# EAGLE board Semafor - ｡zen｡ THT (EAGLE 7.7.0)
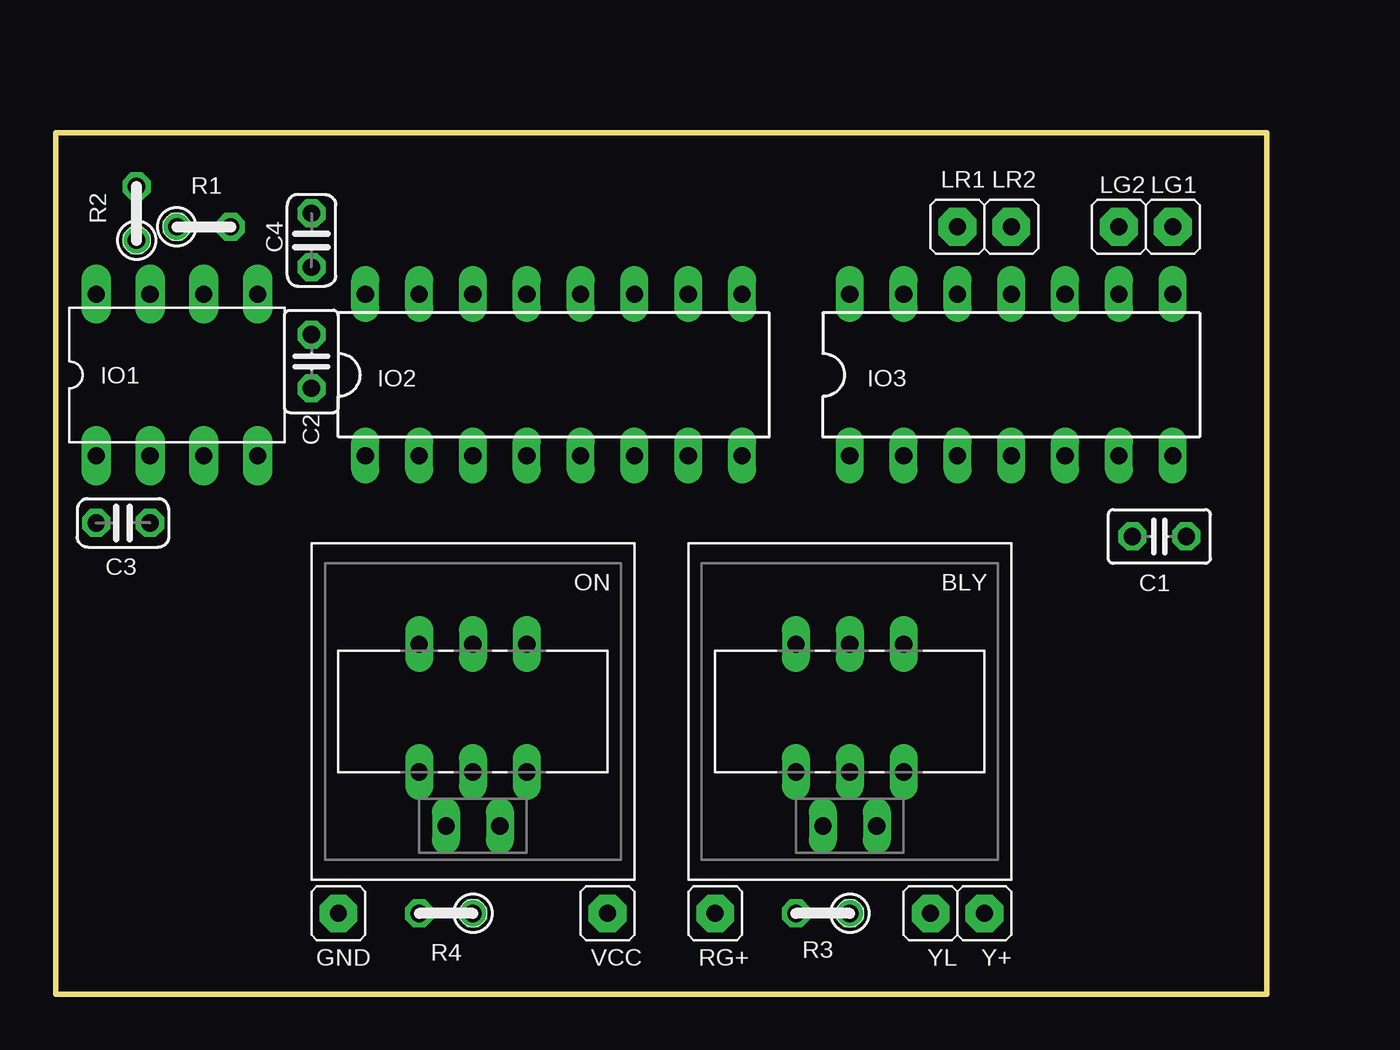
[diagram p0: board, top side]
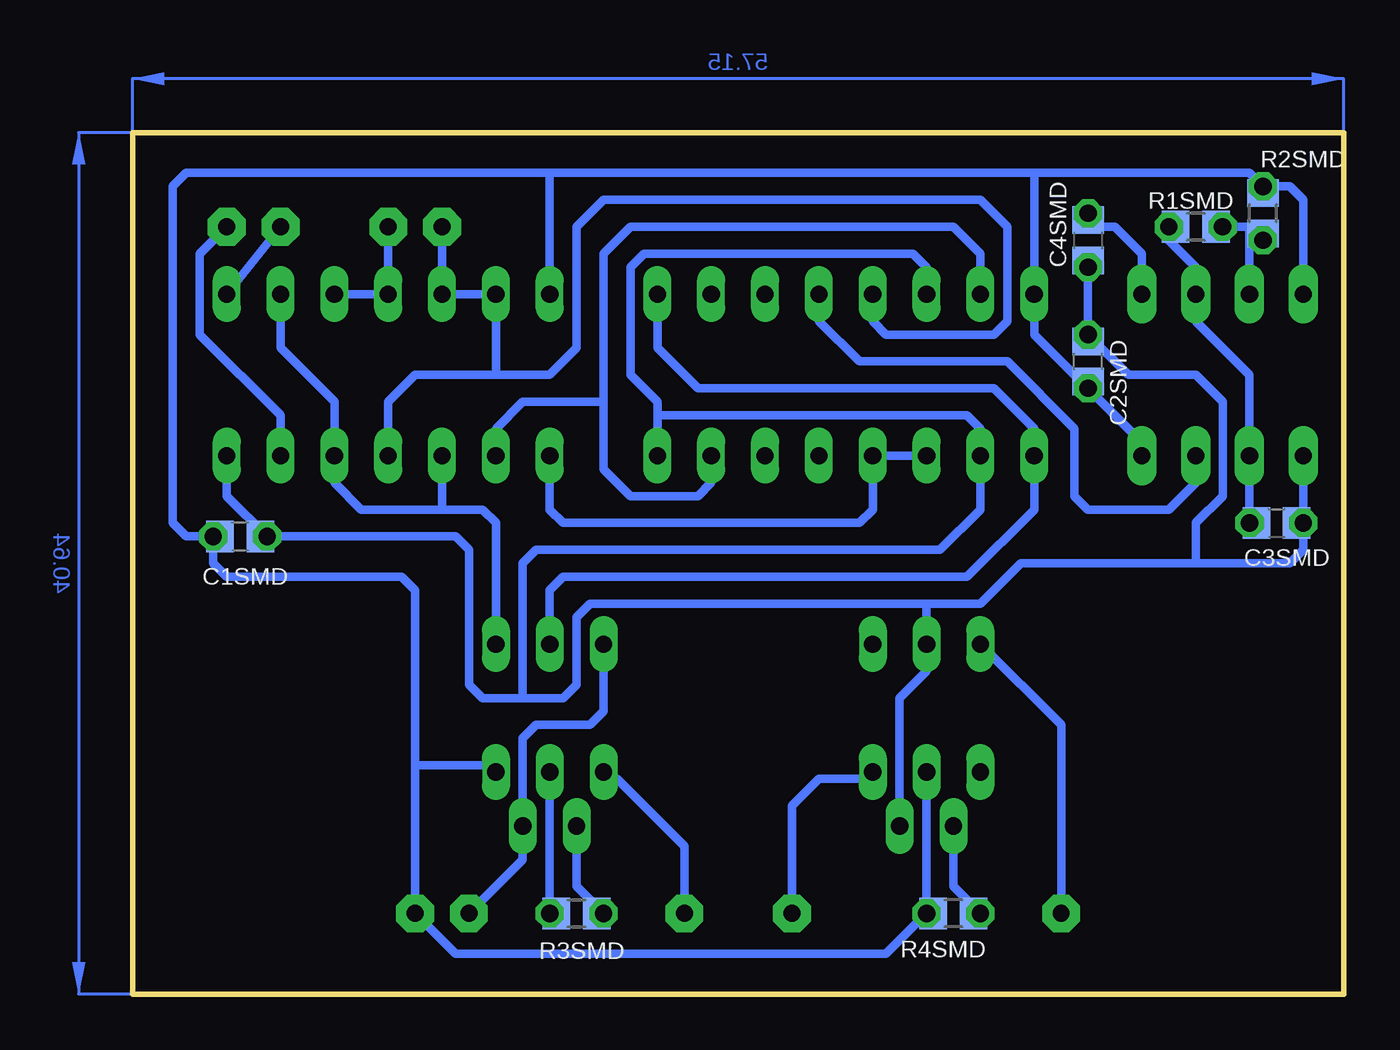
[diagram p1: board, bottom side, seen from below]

Size 57.15 x 40.64 mm. Coordinates in mm from the lower left corner, seen from the top.
Outline: 0,0 57.15,0 57.15,40.64 0,40.64 0,0
Copper layers (1*16): Top 0.035mm / dielectric 1.5mm / Bottom 0.035mm
Design rules "default": minimum track width 10mil, minimum drill 24mil, track to track 8mil, track to pad 8mil, pad to pad 8mil, via to via 8mil, smd to smd 8mil, copper to edge 40mil, drill to drill 8mil, minimum pad ring 10mil, minimum via ring 8mil, stop-mask expansion 4mil, vias tented up to drill 0mil, thermal gap 10mil

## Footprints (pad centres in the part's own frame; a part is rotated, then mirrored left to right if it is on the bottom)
P-0S?B = drill 0.813 pad 1.27 long: 1 2.54,-3.175; 2 0,-3.175; 3 -2.54,-3.175; 4 -2.54,2.857; 5 0,2.857; 6 2.54,2.857; A1 1.27,5.397; K1 -1.27,5.397
C025-025X050 = drill 0.813 octagon: 1 -1.27,0; 2 1.27,0
C0805 = smd 1.3 x 1.5: 1 -0.95,0; 2 0.95,0
C025-024X044 = drill 0.813 octagon: 1 -1.27,0; 2 1.27,0
S1G1_JUM = drill 0.8 pad 1.778 octagon: 1 0,0
DIL8 = drill 0.813 pad 1.4 long: 1 -3.81,-3.81; 2 -1.27,-3.81; 3 1.27,-3.81; 4 3.81,-3.81; 5 3.81,3.81; 6 1.27,3.81; 7 -1.27,3.81; 8 -3.81,3.81
DIL16 = drill 0.813 long: 1 -8.89,-3.81; 2 -6.35,-3.81; 3 -3.81,-3.81; 4 -1.27,-3.81; 5 1.27,-3.81; 6 3.81,-3.81; 7 6.35,-3.81; 8 8.89,-3.81; 9 8.89,3.81; 10 6.35,3.81; 11 3.81,3.81; 12 1.27,3.81; 13 -1.27,3.81; 14 -3.81,3.81; 15 -6.35,3.81; 16 -8.89,3.81
DIL14 = drill 0.813 long: 1 -7.62,-3.81; 2 -5.08,-3.81; 3 -2.54,-3.81; 4 0,-3.81; 5 2.54,-3.81; 6 5.08,-3.81; 7 7.62,-3.81; 8 7.62,3.81; 9 5.08,3.81; 10 2.54,3.81; 11 0,3.81; 12 -2.54,3.81; 13 -5.08,3.81; 14 -7.62,3.81
0204V = drill 0.813 octagon: 1 -1.27,0; 2 1.27,0
R0805 = smd 1.3 x 1.5: 1 -0.95,0; 2 0.95,0

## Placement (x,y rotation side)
BLY  [P-0S?B]  37.47,13.34 180 top
C1  [C025-025X050]  52.07,21.59 180 top
C1SMD  [C0805]  52.07,21.59 0 bottom
C2  [C025-025X050]  12.06,29.84 90 top
C2SMD  [C0805]  12.06,29.84 90 bottom
C3  [C025-024X044]  3.17,22.23 180 top
C3SMD  [C0805]  3.17,22.23 0 bottom
C4  [C025-024X044]  12.06,35.56 270 top
C4SMD  [C0805]  12.06,35.56 270 bottom
GND  [S1G1_JUM]  13.34,3.81 0 top
IO1  CMOS555  [DIL8]  5.71,29.21 0 top
IO2  74HCT390  [DIL16]  23.5,29.21 0 top
IO3  74HCT00  [DIL14]  45.09,29.21 0 top
LG1  [S1G1_JUM]  52.7,36.2 0 top
LG2  [S1G1_JUM]  50.16,36.2 0 top
LR1  [S1G1_JUM]  42.55,36.2 0 top
LR2  [S1G1_JUM]  45.09,36.2 0 top
ON  [P-0S?B]  19.68,13.34 180 top
R1  [0204V]  6.99,36.2 0 top
R1SMD  [R0805]  6.99,36.2 180 bottom
R2  [0204V]  3.81,36.83 90 top
R2SMD  [R0805]  3.81,36.83 90 bottom
R3  [0204V]  36.2,3.81 180 top
R3SMD  [R0805]  36.2,3.81 0 bottom
R4  [0204V]  18.41,3.81 180 top
R4SMD  [R0805]  18.41,3.81 180 bottom
RG+  [S1G1_JUM]  31.11,3.81 0 top
VCC  [S1G1_JUM]  26.04,3.81 0 top
Y+  [S1G1_JUM]  43.81,3.81 0 top
YL  [S1G1_JUM]  41.27,3.81 0 top

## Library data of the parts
BLY ON = #PaJa_prepinace
C1 C1SMD C2 C2SMD C3 C3SMD C4 C4SMD R1 R1SMD R2 R2SMD R3 R3SMD R4 R4SMD = rcl
GND LG1 LG2 LR1 LR2 RG+ VCC Y+ YL = #PaJa_konektory
IO1 = #PaJa_31
IO2 IO3 = 74xx-eu

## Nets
N$1: ON.A1 R4.2 R4SMD.1
N$2: BLY.6 RG+.1
N$4: GND.1 ON.1
N$5: ON.4 VCC.1
N$6: BLY.A1 R3.2 R3SMD.2
N$8: BLY.1 BLY.K1 YL.1
N$9: IO2.13 IO3.4 IO3.12 IO3.13 LR1.1
N$10: IO2.7 IO2.15 IO3.2
N$11: IO2.3 IO2.4 IO3.1
N$12: BLY.3 IO3.3 IO3.5 IO3.9
N$13: BLY.2 IO2.1 IO2.9
N$14: C1.2 C1SMD.2 C2.2 C2SMD.2 C3.2 C3SMD.2 C4.2 C4SMD.2 IO1.1 IO2.2 IO2.8 IO2.14 IO3.7 ON.2 ON.K1
N$15: IO1.3 IO2.12
N$16: C4.1 C4SMD.1 IO1.5
N$17: C3.1 C3SMD.1 IO1.2 IO1.6 R1.2 R1SMD.2
N$18: IO1.7 R1.1 R1SMD.1 R2.1 R2SMD.1
N$19: IO3.10 IO3.11 LR2.1
N$20: IO3.6 LG1.1
N$21: BLY.5 R3.1 R3SMD.1
N$27: IO3.8 LG2.1
N$28: BLY.4 C1.1 C1SMD.1 C2.1 C2SMD.1 IO1.4 IO1.8 IO2.16 IO3.14 ON.5 R2.2 R2SMD.2 R4.1 R4SMD.2 Y+.1

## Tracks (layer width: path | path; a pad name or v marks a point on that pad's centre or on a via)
N$1
  Bottom 0.406: ON.A1 18.41,5.08 R4.2 R4SMD.1
N$2
  Bottom 0.406: RG+.1 31.11,6.99 34.29,10.16 34.61,10.16 BLY.6
N$4
  Bottom 0.406: GND.1 13.34,12.7 ON.1
N$5
  Bottom 0.406: VCC.1 26.04,8.89 24.77,10.16 22.54,10.16 ON.4
N$6
  Bottom 0.406: BLY.A1 36.2,5.08 R3.2 R3SMD.2
N$8
  Bottom 0.406: BLY.1 34.92,13.34 35.56,12.7 38.1,12.7 38.73,12.06 BLY.K1 38.73,6.35 YL.1
N$9
  Bottom 0.406: IO2.13 22.23,31.75 21.59,31.11 16.51,31.11 15.88,31.75 15.88,36.2 17.14,37.47 34.92,37.47 36.2,36.2 36.2,30.48 37.47,29.21 40.01,29.21 | 40.01,29.21 43.81,29.21 45.09,27.94 IO3.4 | 40.01,29.21 IO3.13 IO3.12 LR1.1
N$10
  Bottom 0.406: IO2.15 17.14,34.92 18.41,36.2 33.66,36.2 34.92,34.92 34.92,27.94 | 34.92,27.94 34.92,24.77 33.66,23.5 30.48,23.5 29.84,24.13 IO2.7 | IO3.2 40.01,26.67 38.73,27.94 34.92,27.94
N$11
  Bottom 0.406: IO2.3 IO2.4 22.23,22.86 22.86,22.23 36.83,22.23 37.47,22.86 IO3.1
N$12
  Bottom 0.406: IO3.9 50.16,30.48 47.62,27.94 IO3.5 47.62,24.13 46.35,22.86 42.55,22.86 | BLY.3 40.01,22.23 40.64,22.86 42.55,22.86 | IO3.3 42.55,22.86
N$13
  Bottom 0.406: IO2.9 32.38,30.48 30.48,28.57 16.51,28.57 14.61,26.67 IO2.1 14.61,22.86 17.78,19.68 36.83,19.68 37.47,19.05 BLY.2
N$14
  Bottom 0.406: IO2.14 19.68,34.29 20.32,34.92 33.02,34.92 33.66,34.29 33.66,29.21 32.38,27.94 32.38,27.3 | 32.38,27.3 IO2.8 | 32.38,27.3 17.78,27.3 17.14,26.67 IO2.2 17.14,22.86 19.05,20.95 38.1,20.95 38.73,20.32 38.73,13.97 | IO1.1 C3.2 | ON.K1 20.95,13.97 19.68,15.24 ON.2 19.68,18.41 | 38.73,13.97 36.83,13.97 36.2,14.61 36.2,17.78 35.56,18.41 19.68,18.41 | 19.68,18.41 17.14,18.41 15.24,20.32 6.99,20.32 | C2.2 C4.2 C4SMD.2 | C2.2 10.16,29.21 6.99,29.21 5.71,27.94 5.71,23.5 6.99,22.23 6.99,20.32 | 38.73,13.97 40.64,13.97 41.27,14.61 41.27,20.95 41.91,21.59 C1.2 | IO3.7 52.7,23.5 C1.2 | C2SMD.2 C2.2 | C3.2 C3SMD.2 | C1SMD.2 C1.2 | C3.2 1.91,20.95 2.54,20.32 6.99,20.32
N$15
  Bottom 0.406: IO1.3 6.99,24.13 8.26,22.86 12.06,22.86 12.7,23.5 12.7,26.67 15.88,29.84 22.86,29.84 24.77,31.75 IO2.12
N$16
  Bottom 0.406: IO1.5 9.53,34.92 10.79,36.2 11.43,36.2 | 11.43,36.2 11.75,36.2 C4SMD.1 | C4.1 11.43,36.2
N$17
  Bottom 0.406: R1SMD.2 R1.2 8.26,35.56 6.99,34.29 IO1.6 6.99,31.75 4.45,29.21 IO1.2 C3.1 C3SMD.1
N$18
  Bottom 0.406: R1SMD.1 R1.1 4.45,36.2 | IO1.7 4.45,36.2 | 3.49,36.2 R2SMD.1 | R2.1 R2SMD.1 | 4.45,36.2 4.12,36.2 R2SMD.1
N$19
  Bottom 0.406: IO3.10 IO3.11 LR2.1
N$20
  Bottom 0.406: IO3.6 50.16,27.3 53.98,31.11 53.98,34.92 LG1.1
N$21
  Bottom 0.406: BLY.5 R3.1 R3SMD.1
N$27
  Bottom 0.406: IO3.8 LG2.1
N$28
  Bottom 0.406: 37.47,38.73 54.61,38.73 55.24,38.1 55.24,22.23 54.61,21.59 C1.1 | 37.47,38.73 14.61,38.73 | 14.61,38.73 IO2.16 14.61,31.11 C2.1 | IO3.14 37.47,38.73 | ON.5 R4.1 | R4.1 21.59,1.91 41.91,1.91 Y+.1 43.81,10.79 | 43.81,10.79 40.32,10.79 BLY.4 | IO1.4 9.53,26.04 C2.1 | IO1.8 1.91,37.47 2.54,38.1 R2.2 | 43.81,10.79 43.81,19.05 44.45,19.68 52.7,19.68 53.34,20.32 C1.1 | C2SMD.1 C2.1 | C1SMD.1 C1.1 | R4.1 R4SMD.2 | 14.61,38.73 4.45,38.73 R2.2 | R2SMD.2 R2.2
(copper drawn outside any net)
  shapes: Bottom area x2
